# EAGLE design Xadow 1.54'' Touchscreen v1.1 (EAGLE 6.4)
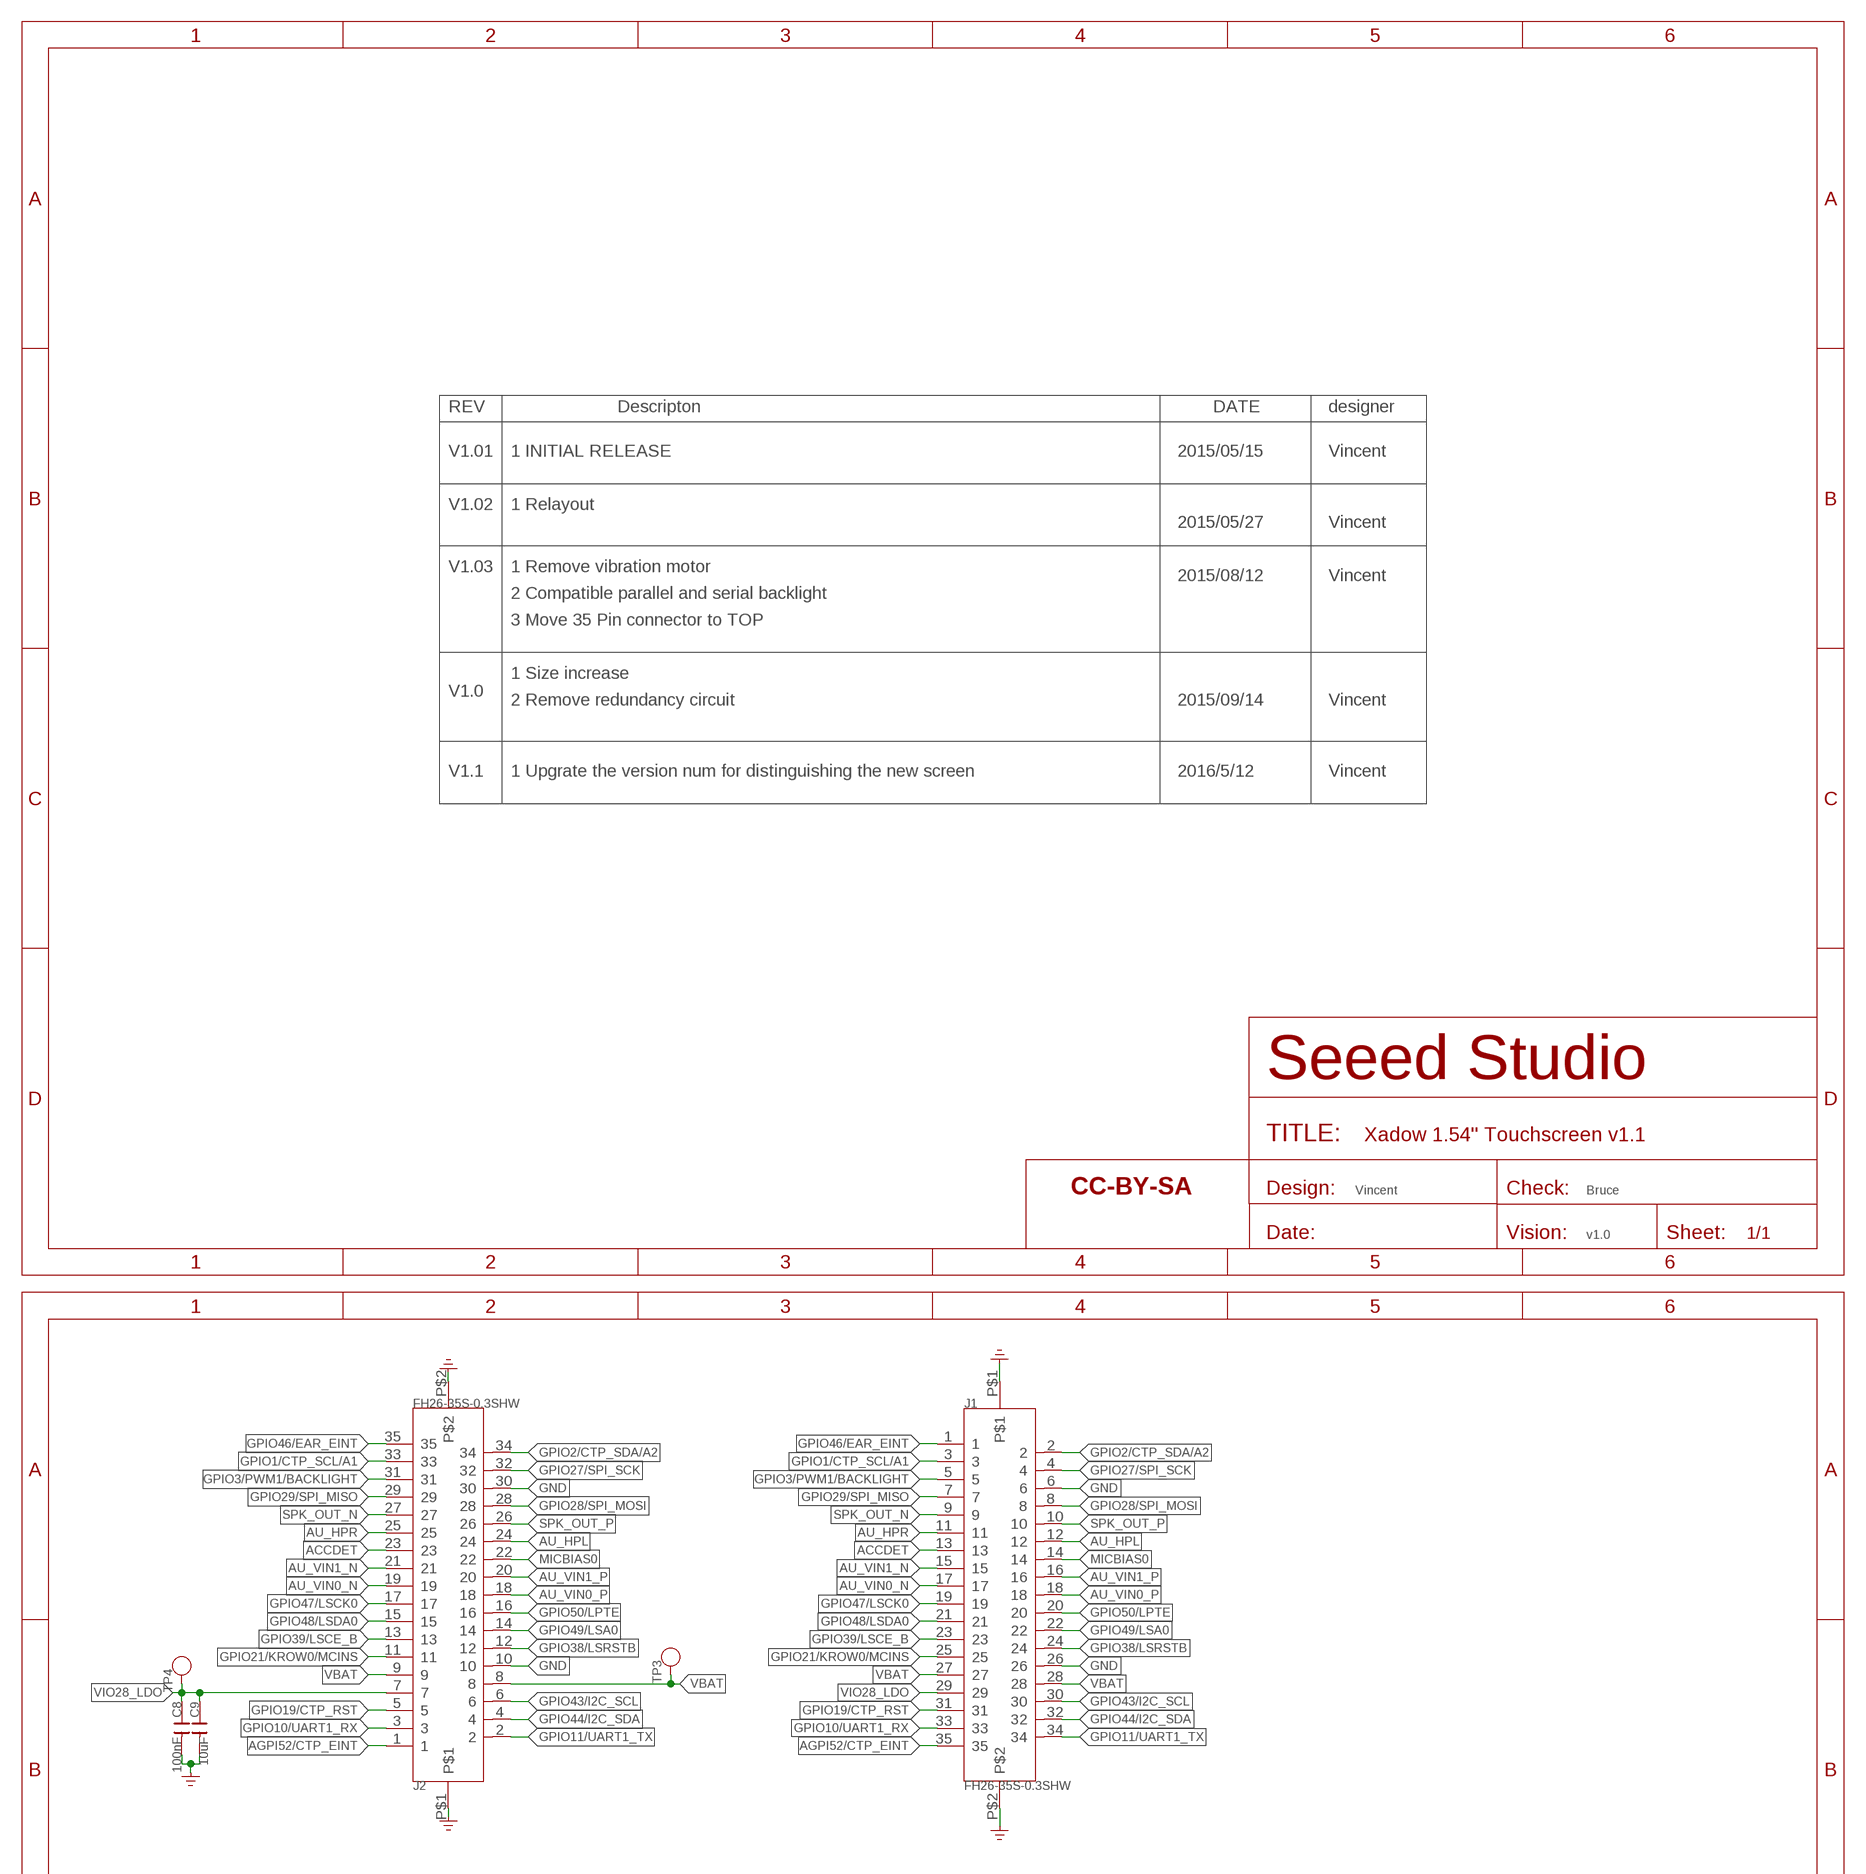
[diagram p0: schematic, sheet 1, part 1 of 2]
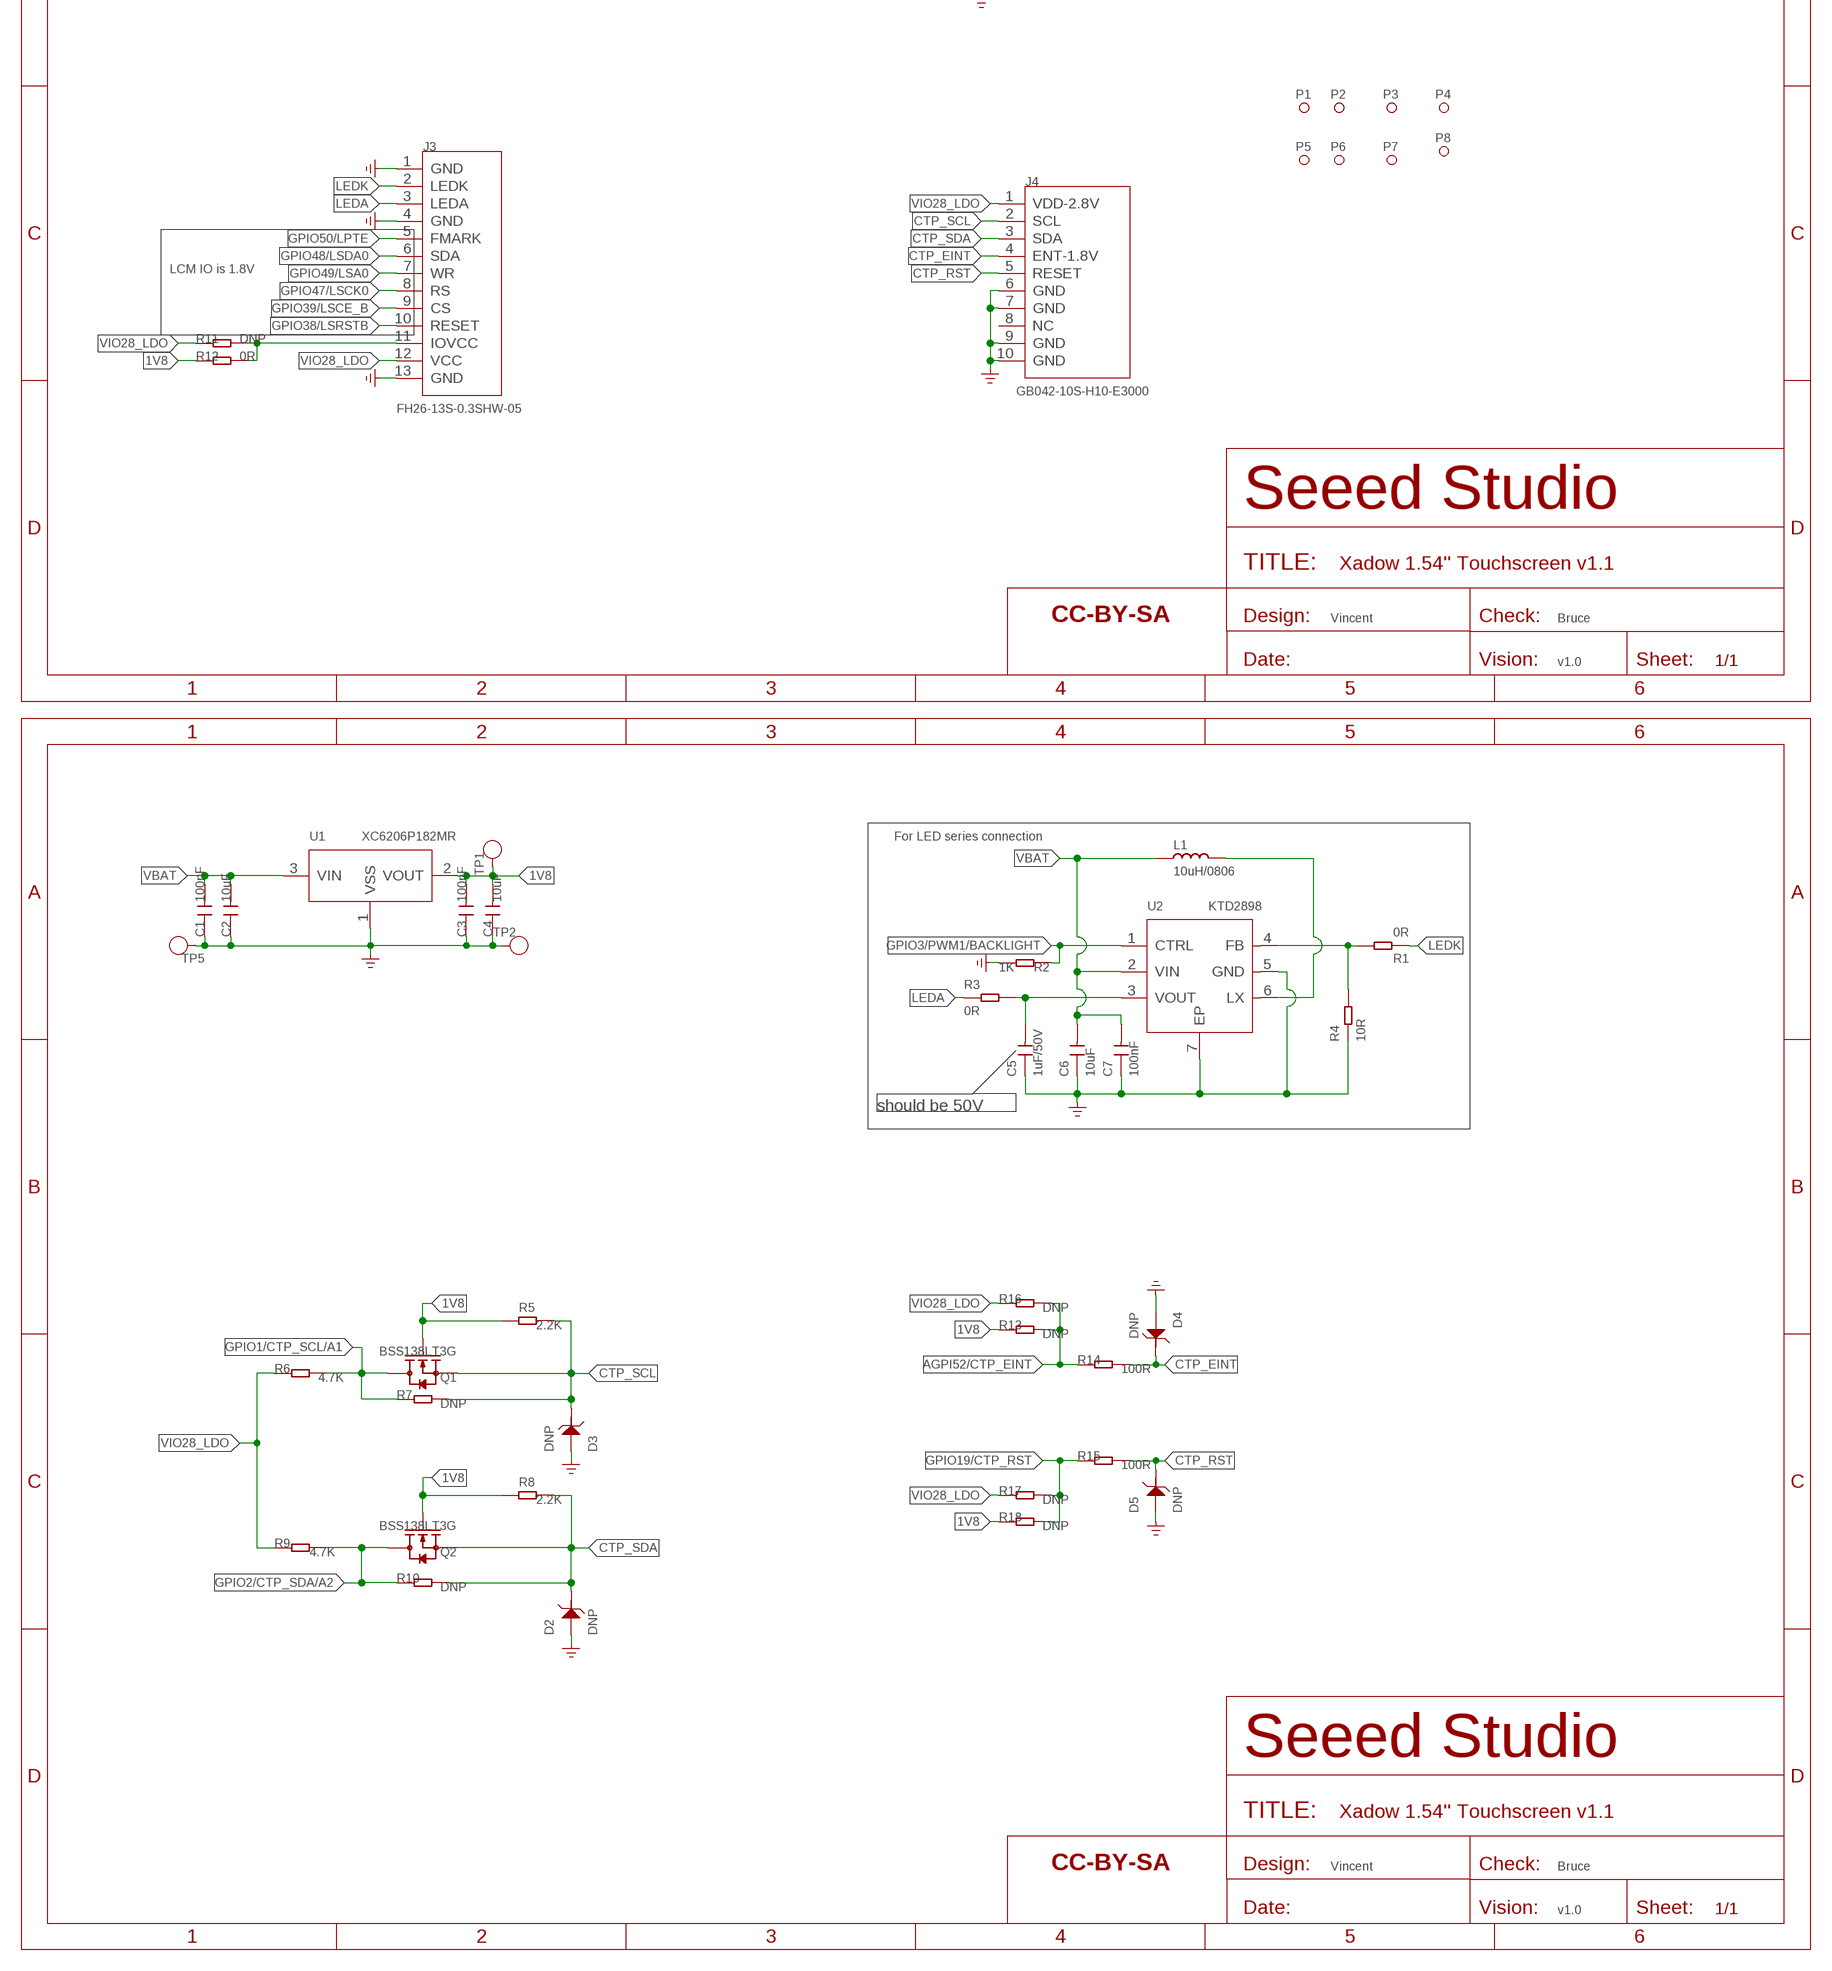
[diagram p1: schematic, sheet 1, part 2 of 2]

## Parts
C1  100nF  CAP-0402  [C0402]
C2  10uF  CAP-0603  [C0603]
C3  100nF  CAP-0402  [C0402]
C4  10uF  CAP-0603  [C0603]
C5  1uF/50V  CAP-0603  [C0603]
C6  10uF  CAP-0603  [C0603]
C7  100nF  CAP-0402  [C0402]
C8  100nF  CAP-0402  [C0402]
C9  10uF  CAP-0603  [C0603]
D2  DNP  D-ESD-2P'DF2S6.8FS'  [SOD-923]
D3  DNP  D-ESD-2P'DF2S6.8FS'  [SOD-923]
D4  DNP  D-ESD-2P'DF2S6.8FS'  [SOD-923]
D5  DNP  D-ESD-2P'DF2S6.8FS'  [SOD-923]
FR1  SEEEDSTUDIO-OPEN-SCH-FRAME  [SEEEDSTUDIO-PCB-FRAME]
FR2  SEEEDSTUDIO-OPEN-SCH-FRAME  [SEEEDSTUDIO-PCB-FRAME]
FR3  SEEEDSTUDIO-OPEN-SCH-FRAME  [SEEEDSTUDIO-PCB-FRAME]
J1  FH26-35S-0.3SHW  FPC-CONNECTER-35P(FH26W-35S-0.3SHW(10))  [FPC35-SMD-0.3(FH26W)]
J2  FH26-35S-0.3SHW  FPC-CONNECTER-35P(FH26W-35S-0.3SHW(10))  [FPC35-SMD-0.3(FH26W)]
J3  FH26-13S-0.3SHW-05  [13P-SMD-FH26-13S-0.3HW]
J4  GB042-10S-H10-E3000  [10P-SMD-GB042-10S-H10]
L1  10uH/0806  INDUCTOR/FERRITE-BEAD'0806'  [L0806]
P1  MARK-1.0'ANNULAR'  [ROUND-MARK-1.0]
P2  MARK-1.0'ANNULAR'  [ROUND-MARK-1.0]
P3  MARK-1.0'ANNULAR'  [ROUND-MARK-1.0]
P4  MARK-1.0'ANNULAR'  [ROUND-MARK-1.0]
P5  MARK-1.0'ANNULAR'  [ROUND-MARK-1.0]
P6  MARK-1.0'ANNULAR'  [ROUND-MARK-1.0]
P7  MARK-1.0'ANNULAR'  [ROUND-MARK-1.0]
P8  MARK-1.0'ANNULAR'  [ROUND-MARK-1.0]
Q1  BSS138LT3G  MOSFET-N'SOT23'  [SOT-23]
Q2  BSS138LT3G  MOSFET-N'SOT23'  [SOT-23]
R1  0R  RES-0402  [R0402]
R2  1K  RES-0402  [R0402]
R3  0R  RES-0402  [R0402]
R4  10R  RES-0402  [R0402]
R5  2.2K  RES-0402  [R0402]
R6  4.7K  RES-0402  [R0402]
R7  DNP  RES-0402  [R0402]
R8  2.2K  RES-0402  [R0402]
R9  4.7K  RES-0402  [R0402]
R10  DNP  RES-0402  [R0402]
R11  DNP  RES-0402  [R0402]
R12  0R  RES-0402  [R0402]
R13  DNP  RES-0402  [R0402]
R14  100R  RES-0402  [R0402]
R15  100R  RES-0402  [R0402]
R16  DNP  RES-0402  [R0402]
R17  DNP  RES-0402  [R0402]
R18  DNP  RES-0402  [R0402]
TP1  TEST-POINT'4545'  [TP-D45MIL]
TP2  TEST-POINT'4545'  [TP-D45MIL]
TP3  TEST-POINT'4545'  [TP-D45MIL]
TP4  TEST-POINT'4545'  [TP-D45MIL]
TP5  TEST-POINT'4545'  [TP-D45MIL]
U1  XC6206P182MR  PMIC-XC6206PMR  [SOT-23]
U2  KTD2898  [6P-SMD-KTD2898]

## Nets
1V8: C3.2 C4.2 Q1.1(G) Q2.1(G) R5.1 R8.1 R12.1 R13.1 R18.1 TP1.T U1.2(VOUT)
ACCDET: J1.13 J2.23
AGPI52/CTP_EINT: J1.35 J2.1 R13.2 R14.1 R16.2
AU_HPL: J1.12 J2.24
AU_HPR: J1.11 J2.25
AU_VIN0_N: J1.17 J2.19
AU_VIN0_P: J1.18 J2.18
AU_VIN1_N: J1.15 J2.21
AU_VIN1_P: J1.16 J2.20
CTP_EINT: D4.1 J4.4(ENT-1.8V) R14.2
CTP_RST: D5.1 J4.5(RESET) R15.2
CTP_SCL: D3.1 J4.2(SCL) Q1.2(S) R5.2 R7.2
CTP_SDA: D2.1 J4.3(SDA) Q2.2(S) R8.2 R10.2
GND: C1.1 C2.1 C3.1 C4.1 C5.1 C6.1 C7.1 C8.2 C9.2 D2.2 D3.2 D4.2 D5.2 J1.6 J1.26 J1.P$1 J1.P$2 J2.10 J2.30 J2.P$1 J2.P$2 J3.1(GND) J3.4(GND) J3.13(GND) J4.6(GND) J4.7(GND) J4.9(GND) J4.10(GND) R2.1 R4.1 TP2.T TP5.T U1.1(VSS) U2.5(GND) U2.7(EP) ; supply symbol labelled GND_POWER
GPIO1/CTP_SCL/A1: J1.3 J2.33 Q1.3(D) R6.2 R7.1
GPIO2/CTP_SDA/A2: J1.2 J2.34 Q2.3(D) R9.2 R10.1
GPIO3/PWM1/BACKLIGHT: J1.5 J2.31 R2.2 U2.1(CTRL)
GPIO10/UART1_RX: J1.33 J2.3
GPIO11/UART1_TX: J1.34 J2.2
GPIO19/CTP_RST: J1.31 J2.5 R15.1 R17.2 R18.2
GPIO21/KROW0/MCINS: J1.25 J2.11
GPIO27/SPI_SCK: J1.4 J2.32
GPIO28/SPI_MOSI: J1.8 J2.28
GPIO29/SPI_MISO: J1.7 J2.29
GPIO38/LSRSTB: J1.24 J2.12 J3.10(RESET)
GPIO39/LSCE_B: J1.23 J2.13 J3.9(CS)
GPIO43/I2C_SCL: J1.30 J2.6
GPIO44/I2C_SDA: J1.32 J2.4
GPIO46/EAR_EINT: J1.1 J2.35
GPIO47/LSCK0: J1.19 J2.17 J3.8(RS)
GPIO48/LSDA0: J1.21 J2.15 J3.6(SDA)
GPIO49/LSA0: J1.22 J2.14 J3.7(WR)
GPIO50/LPTE: J1.20 J2.16 J3.5(FMARK)
LEDA: J3.3(LEDA) R3.1
LEDK: J3.2(LEDK) R1.1
MICBIAS0: J1.14 J2.22
N$1: R1.2 R4.2 U2.4(FB)
N$2: C5.2 R3.2 U2.3(VOUT)
N$3: J3.11(IOVCC) R11.2 R12.2
N$5: L1.2 U2.6(LX)
SPK_OUT_N: J1.9 J2.27
SPK_OUT_P: J1.10 J2.26
VBAT: C1.2 C2.2 C6.2 C7.2 J1.27 J1.28 J2.8 J2.9 L1.1 TP3.T U1.3(VIN) U2.2(VIN)
VIO28_LDO: C8.1 C9.1 J1.29 J2.7 J3.12(VCC) J4.1(VDD-2.8V) R6.1 R9.1 R11.1 R16.1 R17.1 TP4.T
Unconnected: J4.8(NC)

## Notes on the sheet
- REV | Descripton | DATE | designer
- V1.01 | 1 INITIAL RELEASE | 2015/05/15 | Vincent
- V1.02 | 1 Relayout
- 2015/05/27 | Vincent
- V1.03 | 1 Remove vibration motor
- 2015/08/12 | Vincent
- 2 Compatible parallel and serial backlight
- 3 Move 35 Pin connector to TOP
- 1 Size increase
- V1.0
- 2 Remove redundancy circuit | 2015/09/14 | Vincent
- V1.1 | 1 Upgrate the version num for distinguishing the new screen | 2016/5/12 | Vincent
- Vincent | Bruce
- v1.0
- LCM IO is 1.8V
- Vincent | Bruce
- v1.0
- For LED series connection
- should be 50V
- Vincent | Bruce
- v1.0

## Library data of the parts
C1-C9 = Discrete-new:CAP: Ceramic Capacitors
D2-D5 = Discrete-new:D-ESD-2P: SOD-923:304060009;SOD-123:304060001
FR1-FR3 = moudle-new:SEEEDSTUDIO-OPEN-SCH-FRAME
J1 J2 = template:FPC-CONNECTER-35P(FH26W-35S-0.3SHW(10))
J3 = template:FH26-13S-0.3SHW-05
J4 = template:GB042-10S-H10-E3000
L1 = Discrete-new:INDUCTOR/FERRITE-BEAD
P1-P8 = Discrete-new:MARK-1.0; PARTNO: DNP
Q1 Q2 = Discrete-new:MOSFET-N
R1-R18 = Discrete-new:RES
TP1-TP5 = Discrete-new:TEST-POINT; PARTNO: DNP
U1 = IC-new:PMIC-XC6206P: LOW ESR Cap.Compatible Positive Voltage Regulators
U2 = template:KTD2898

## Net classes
0 default: width 0.076 mm, drill 0.102 mm, clearance 0.076 mm

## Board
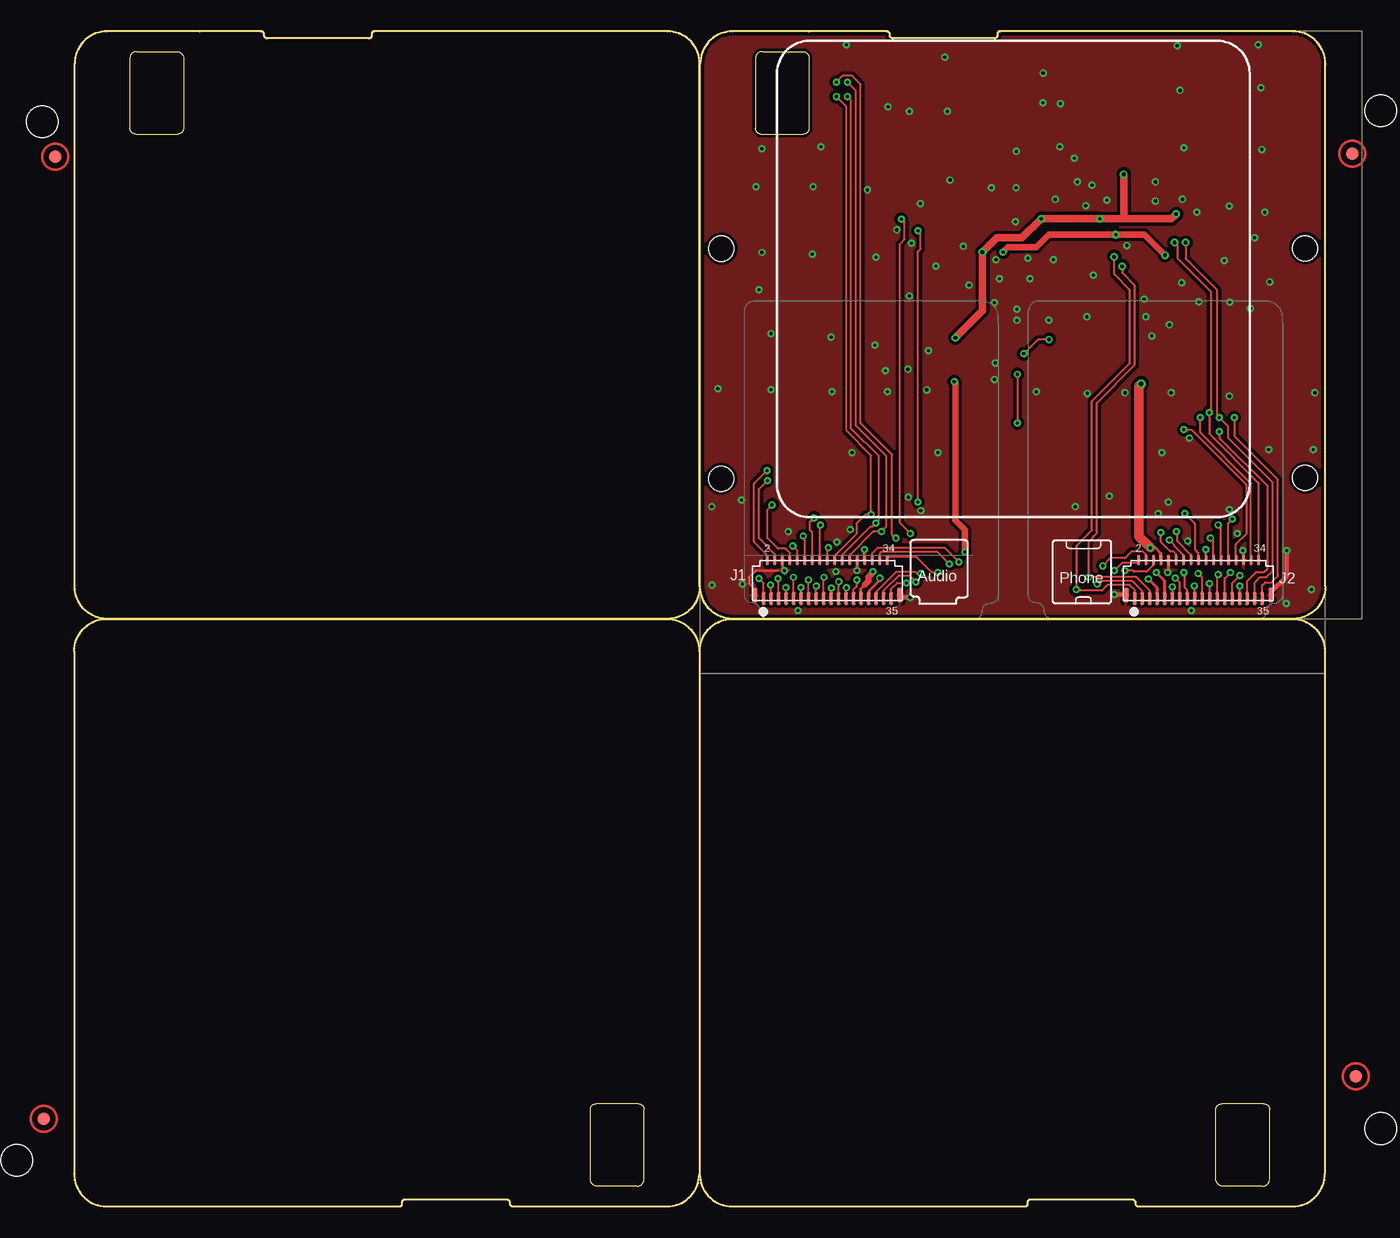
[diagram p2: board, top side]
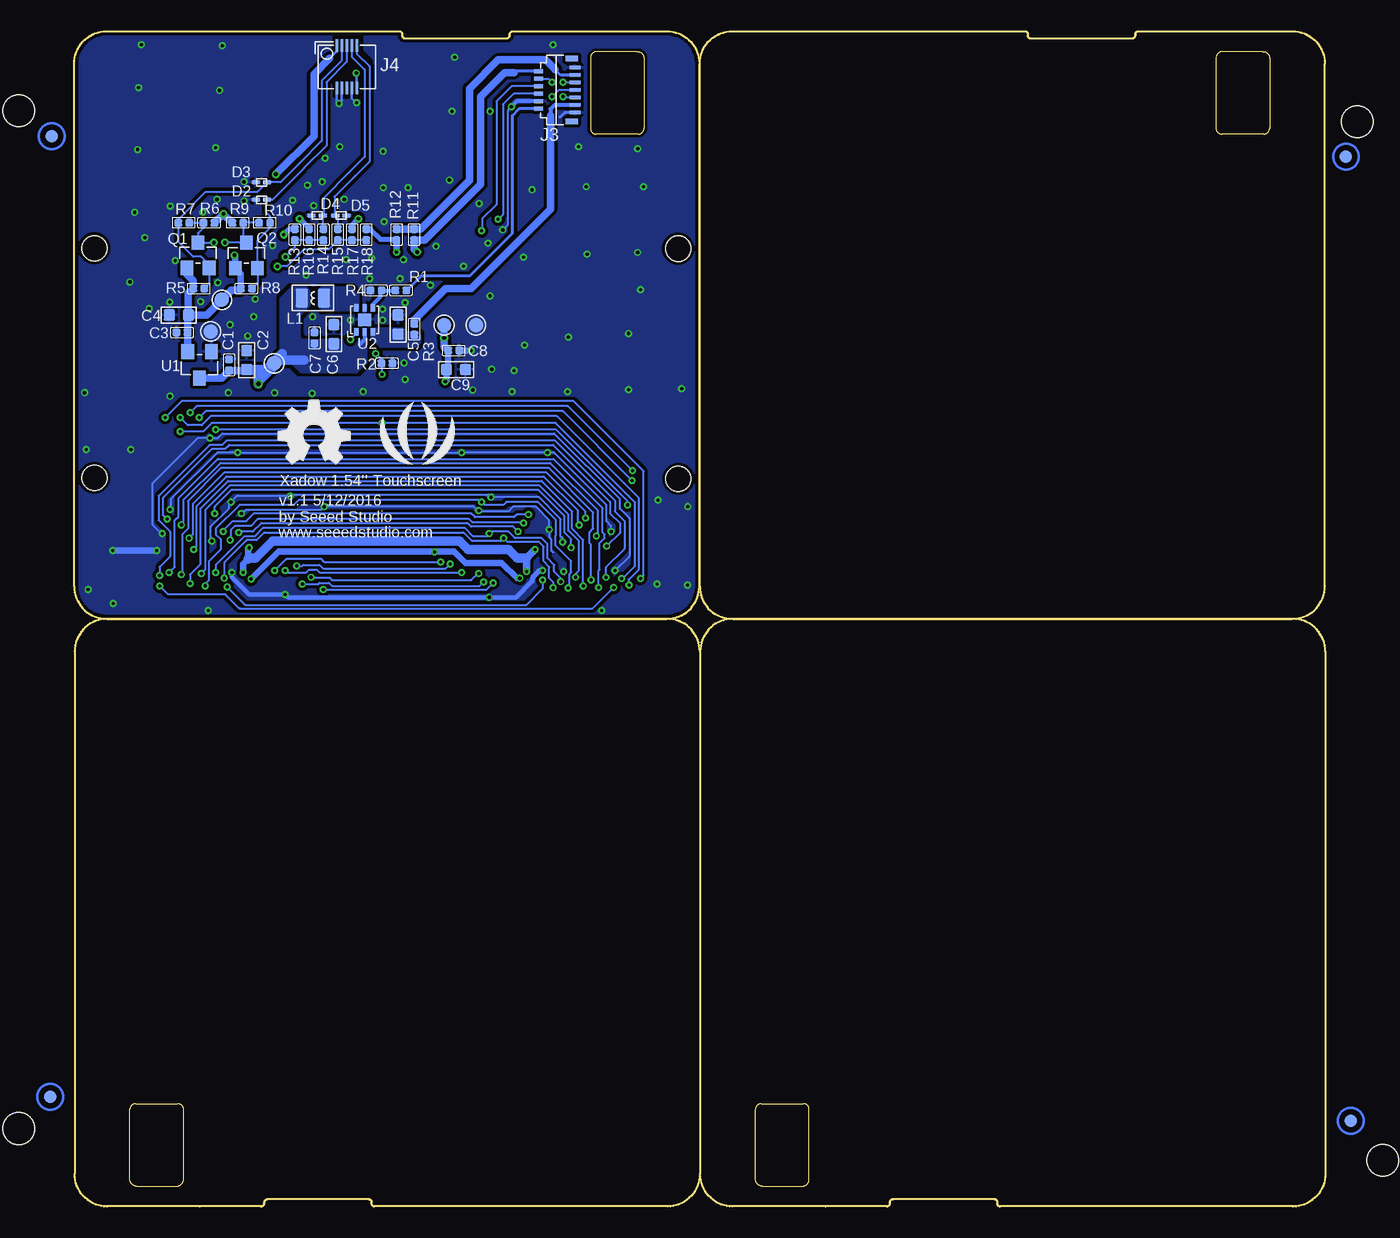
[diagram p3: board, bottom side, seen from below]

Size 100.08 x 94 mm. Coordinates in mm from the lower left corner, seen from the top.
Outline: 104 segments
Copper layers (1*16): Top 0.035mm / dielectric 1.5mm / Bottom 0.035mm
Design rules "SeeedStudio_2layer_DRU_no_angle_20140221 *": minimum track width 6mil, minimum drill 10mil, track to track 6mil, track to pad 6mil, pad to pad 6mil, via to via 6mil, smd to smd 0mil, copper to edge 10mil, drill to drill 10mil, minimum pad ring 10mil, minimum via ring 6mil, stop-mask expansion 2mil, vias tented up to drill 25mil, thermal gap 10mil
Holes 2.03 mm at 51.77,76.62 51.74,58.2 98.46,58.28 98.46,76.64
Holes 2.54 mm at -2.54,86.75 -4.57,3.69 104.52,6.23 104.52,87.64

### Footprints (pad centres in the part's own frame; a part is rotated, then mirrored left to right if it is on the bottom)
C0402 = smd 0.635 x 0.635: 1 0,0.445; 2 0,-0.445
C0603 = smd 0.889 x 0.889: 1 0,0.762; 2 0,-0.762
SOD-923 = smd 0.7 x 0.3: 1 -0.45,0; 2 0.45,0
FPC35-SMD-0.3(FH26W) = smd 0.3 x 1: 1 -5.1,-1.551; 3 -4.5,-1.551; 5 -3.9,-1.551; 7 -3.3,-1.551; 9 -2.7,-1.551; 11 -2.1,-1.551; 13 -1.5,-1.551; 15 -0.9,-1.551; 17 -0.3,-1.551; 19 0.3,-1.551; 21 0.9,-1.551; 23 1.5,-1.551; 25 2.1,-1.551; 27 2.7,-1.551; 29 3.3,-1.551; 31 3.9,-1.551; 33 4.5,-1.551; 35 5.1,-1.551 | smd 0.254 x 0.851: 2 -4.8,1.524; 4 -4.2,1.524; 6 -3.6,1.524; 8 -3,1.524; 10 -2.4,1.524; 12 -1.8,1.524; 14 -1.2,1.524; 16 -0.6,1.524; 18 0,1.524; 20 0.6,1.524; 22 1.2,1.524; 24 1.8,1.524; 26 2.4,1.524; 28 3,1.524; 30 3.6,1.524; 32 4.2,1.524; 34 4.8,1.524 | smd 0.4 x 1.15: P$1 5.8,-1.276; P$2 -5.8,-1.276
13P-SMD-FH26-13S-0.3HW = smd 0.3 x 0.85: 1 -1.8,-1.462; 3 -1.2,-1.462; 5 -0.6,-1.462; 7 0,-1.462; 9 0.6,-1.462; 11 1.2,-1.462; 13 1.8,-1.462 | smd 0.3 x 0.7: 2 -1.5,1.462; 4 -0.9,1.462; 6 -0.3,1.462; 8 0.3,1.462; 10 0.9,1.462; 12 1.5,1.462 | smd 0.45 x 1: 14 2.525,-1.188; 15 -2.525,-1.188
10P-SMD-GB042-10S-H10 = smd 0.23 x 1: 1 -0.8,1.7; 2 -0.4,1.7; 3 0,1.7; 4 0.4,1.7; 5 0.8,1.7; 6 0.8,-1.7; 7 0.4,-1.7; 8 0,-1.7; 9 -0.4,-1.7; 10 -0.8,-1.7
L0806 = smd 1.016 x 1.524: 1 -0.889,0; 2 0.889,0
ROUND-MARK-1.0 = smd 1.016 x 1.016: P$1 0,0
SOT-23 = smd 1.016 x 1.143: 1 -0.889,-1.016; 2 0.889,-1.016; 3 0,1.016
R0402 = smd 0.635 x 0.635: 1 0,0.445; 2 0,-0.445
TP-D45MIL = smd 1.143 x 1.143: T 0,0
SOT-23' = smd 1.016 x 1.2: 1 -0.95,-1.06; 2 0.95,-1.06; 3 0,1.06
6P-SMD-KTD2898 = smd 0.35 x 0.58: 1 -0.65,-0.96; 2 0,-0.96; 3 0.65,-0.96; 4 0.65,0.96; 5 0,0.96; 6 -0.65,0.96 | smd 1 x 1: 7 0,0

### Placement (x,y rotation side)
C1  87.68,67.31 0 bottom
C2  86.28,67.69 0 bottom
C3  91.45,69.91 90 bottom
C4  91.7,71.31 90 bottom
C5  74.17,70.54 0 bottom
C6  79.3,69.77 0 bottom
C7  80.85,69.47 0 bottom
C8  69.72,68.46 90 bottom
C9  69.54,66.94 90 bottom
D2  85.09,80.53 180 bottom
D3  85.09,81.92 180 bottom
D4  80.64,79.26 180 bottom
D5  78.74,79.26 0 bottom
FR1  not placed on the board
FR2  not placed on the board
FR3  not placed on the board
J1  60.24,50.17 0 top
J2  89.92,50.17 0 top
J3  61.47,89.3 90 bottom
J4  78.26,91.15 0 bottom
L1  80.98,72.66 0 bottom
P1  101.98,8.77 0 bottom
P2  -2.03,6.87 0 bottom
P3  -1.65,83.96 0 bottom
P4  101.85,85.61 0 bottom
P5  -2.41,6.99 0 top
P6  102.49,10.42 0 top
P7  102.23,84.21 0 top
P8  -1.52,83.96 0 top
Q1  90.17,76.08 0 bottom
Q2  86.3,76.08 0 bottom
R1  73.95,73.27 270 bottom
R2  75.06,67.45 270 bottom
R3  72.88,70.17 0 bottom
R4  75.93,73.27 90 bottom
R5  90.11,73.42 90 bottom
R6  89.29,78.69 270 bottom
R7  91.31,78.69 270 bottom
R8  86.3,73.42 90 bottom
R9  86.99,78.69 90 bottom
R10  84.84,78.69 90 bottom
R11  72.9,77.73 180 bottom
R12  74.3,77.73 180 bottom
R13  82.42,77.73 0 bottom
R14  80.14,77.73 180 bottom
R15  78.99,77.73 180 bottom
R16  81.28,77.73 0 bottom
R17  77.85,77.73 0 bottom
R18  76.71,77.73 0 bottom
TP1  88.27,72.53 0 bottom
TP2  89.15,69.99 0 bottom
TP3  84.07,67.45 0 bottom
TP4  70.48,70.5 0 bottom
TP5  67.94,70.5 0 bottom
U1  XC6206P182MR  [SOT-23']  90.04,67.32 180 bottom
U2  76.84,70.92 0 bottom
U$18  [OSHW_FILLX200_NOTEXT]  83.73,59.41 0 bottom
U$20  [SEEED-SILK-280*268MIL]  72.63,61.06 0 bottom

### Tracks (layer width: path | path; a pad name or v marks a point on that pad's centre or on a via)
1V8  (via drill 0.25 pad 0.51, 0.25 pad 0.61, 0.3)
  Top 0.508: v74.3,76.34 74.68,76.72 76.96,76.72 77.98,77.73 v83.31,77.73 85.6,77.73 v87.25,76.08
  Bottom 0.406: R13.1 82.87,78.18 v83.31,77.73 | R18.1 76.39,78.18 75.56,77.35 74.36,77.35 R12.1
  Bottom 0.508: R8.1 86.74,74.61 Q2.1 87.19,76.02 v87.25,76.08 | R12.1 v74.3,76.34
  Bottom 0.61: Q1.1 91.06,74.56 90.55,74.05 R5.1 90.94,73.03 C4.2 | C4.2 89.49,71.31 TP1.T 87.57,73.23 87.5,73.29 86.87,73.29 R8.1 | U1.2 90.99,69.9 C3.2 91,71.24 C4.2
ACCDET  (via drill 0.25 pad 0.51)
  Top 0.152: J2.23 91.42,50.48 v91.5,50.56 | J1.13 v58.74,50.12
  Bottom 0.152: v58.74,50.12 58.74,52.94 58.87,53.07 58.87,53.91 58.57,54.21 58.57,55.51 62.15,59.09 88.3,59.09 90.96,56.42 90.96,54.21 91.42,53.76 91.42,50.63 v91.5,50.56
AGPI52/CTP_EINT  (via drill 0.25 pad 0.51, 0.3)
  Top 0.152: J1.35 65.34,49.38 65.83,49.87 v66.57,49.87 | J2.1 84.82,49.31 84.41,49.72 82.66,49.72 82.2,49.26 80.22,49.26 v80.14,49.34 80.14,52.84 80.83,53.53 81.41,54.11 81.41,64.4 84.45,67.45 84.45,73.29 83.19,74.56 v83.19,75.96
  Bottom 0.152: v66.57,49.87 67.1,49.34 v80.14,49.34 | R14.1 R16.2 R13.2 82.42,76.72 v83.19,75.96
AU_HPL  (via drill 0.25 pad 0.51)
  Top 0.152: J1.12 58.44,53.5 v58.31,53.63 | J2.24 91.72,54.29 v91.5,54.52
  Bottom 0.152: v91.5,54.52 91.34,54.67 91.34,56.5 88.37,59.47 62,59.47 58.19,55.66 58.19,53.91 58.31,53.78 v58.31,53.63
AU_HPR  (via drill 0.25 pad 0.51)
  Top 0.152: J1.11 58.14,49.51 v58.13,49.52 | 92.03,48.63 J2.25 92.02,50.24 v92.49,50.71
  Bottom 0.152: v92.49,50.71 92.03,51.17 92.03,54.9 91.73,55.2 91.73,56.64 88.58,59.79 61.75,59.79 57.8,55.84 57.8,53.91 57.65,53.76 57.65,53.45 58.03,53.07 58.03,50.94 58.13,50.84 v58.13,49.52
AU_VIN0_N  (via drill 0.25 pad 0.51)
  Top 0.152: J1.17 59.94,50.31 v59.96,50.33 | J2.19 90.22,50.31 v89.9,50.63
  Bottom 0.152: v89.9,50.63 89.59,50.94 89.59,55.71 87.61,57.7 62.9,57.7 60.55,55.34 60.55,54.06 59.71,53.22 59.71,50.86 59.96,50.61 v59.96,50.33
AU_VIN0_P  (via drill 0.25 pad 0.51)
  Top 0.152: J1.18 60.24,52.61 v60.32,52.69 | J2.18 89.92,52.28 89.67,52.54 89.67,54.59 v88.83,55.43
  Bottom 0.152: v60.32,52.69 60.32,53.38 60.85,53.91 60.85,55.22 62.97,57.34 87.46,57.34 88.83,55.97 v88.83,55.43
AU_VIN1_N  (via drill 0.25 pad 0.51)
  Top 0.152: J1.15 59.34,49.6 v59.35,49.62 | J2.21 90.82,49.81 v90.81,49.82
  Bottom 0.152: v59.35,49.62 59.35,53.33 60.24,54.21 60.24,55.59 62.69,58.03 87.77,58.03 89.97,55.83 89.97,51.39 90.81,50.56 v90.81,49.82
AU_VIN1_P  (via drill 0.25 pad 0.51)
  Top 0.152: J2.20 90.52,52.52 v90.51,52.54 | J1.16 59.64,54.45 v59.68,54.49
  Bottom 0.152: v90.51,52.54 90.28,52.77 90.28,56.01 87.89,58.4 62.52,58.4 59.79,55.66 59.79,54.82 59.68,54.72 v59.68,54.49
CTP_EINT
  Bottom 0.152: J4.4 77.86,91.97 76.83,90.94 76.83,83.96 77.99,82.8 78.11,82.69 80.14,80.66 80.14,79.32 D4.1 80.19,78.24 R14.2
CTP_RST
  Bottom 0.152: J4.5 77.47,92.21 76.45,91.2 76.45,83.58 77.61,82.42 77.72,82.31 79.25,80.78 79.25,79.26 D5.1 arc90 78.99,79.06 R15.2
CTP_SCL
  Bottom 0.152: J4.2 78.67,91.65 80.26,90.05 80.26,85.23 82.04,83.45 82.17,83.32 83.57,81.92 D3.1 85.4,81.16 89.53,81.16 91.75,78.95 R7.2 91.75,77.16 90.55,75.96 89.92,75.96 89.28,75.32 Q1.2 89.28,73.8 R5.2
CTP_SDA
  Bottom 0.152: J4.3 78.27,91.54 79.88,89.93 79.88,84.85 81.66,83.07 81.72,83 84.2,80.53 D2.1 84.71,80.46 84.71,79.51 84.4,79.2 R10.2 84.4,78.3 85.41,77.29 Q2.2 85.41,73.87 R8.2
GND  (via drill 0.25, 0.25 pad 0.51)
  Top 0.152: J1.P$1 | 56.31,50.84 54.48,50.84 53.97,50.33 53.97,49.82 54.38,49.41 54.38,48.97 J1.P$2 | J1.6 56.64,51.03 v56.81,50.86
  Top 0.203: J2.30 93.52,52.42 v93.48,52.46
  Top 0.229: J2.10 87.52,50.77 v87.46,50.71
  Top 0.254: J1.26 62.6,51.66 v62.6,50.86
  Top 0.356: 95.72,48.88 J2.P$1 95.72,49.14 96.98,50.4 v96.98,52.46 | 66.06,48.88 J1.P$1 66.22,48.73 v66.87,48.73 | v83.19,48.96 84.07,48.96 J2.P$2
  Bottom 0.152: 82.73,56.88 v82.81,56.8 | v82.81,56.8 87.08,56.8 v87.53,56.35 87.69,56.2 87.69,55.81 89.14,54.37 89.14,53.38 89.06,53.3 v89.06,53.22 | v82.81,56.8 82.66,56.96 66.95,56.96 v66.72,56.73 62.91,56.73 61.16,54.98 61.16,53.6 61.01,53.45 v61.01,53.15 | v86.7,55.43 86.62,55.43 86.32,55.74 80.3,55.74 v80.07,55.97 79.99,56.04 68.17,56.04 67.79,55.66 v67.71,55.66 67.64,55.59 65.35,55.59 64.97,55.97 63.14,55.97 62.07,54.9 v62.07,54.14 62.07,53.53 61.92,53.38 61.92,52.46 61.77,52.31 | v93.02,53.83 93.1,53.83 93.78,54.52 93.78,57.87 90.2,61.45 v89.21,61.45 88.6,61.45 88.22,61.83 61.69,61.83 56.43,56.58 56.43,55.81 55.67,55.05 55.67,52 v56.81,50.86 | v57.12,53.98 57.12,54.44 57.5,54.82 57.5,56.12 61.69,60.31 v62.22,60.31 v69.08,60.31 v87,60.31 88.6,60.31 92.34,56.58 92.34,55.81 v92.41,55.74 | 65.11,87.94 65.41,87.64 65.41,78.5 v65.79,78.11
  Bottom 0.203: J4.7 77.86,88.66 v77.48,88.28 | J4.6 77.47,90.62 v77.5,90.66 | J4.10 79.06,88.41 v78.87,88.22 78.67,88.43 J4.9
  Bottom 0.254: v65.11,87.97 65.11,87.94 | J3.1 60.84,87.5 61.21,87.13 | 78.67,88.48 78.87,88.28
  Bottom 0.305: J3.4 64.68,88.4 v65.11,87.97
  Bottom 0.356: 63.44,50.02 64.74,48.73 v66.87,48.73 82.96,48.73 v83.19,48.96 86.08,48.96 87.46,50.33 v87.46,50.71
  Bottom 0.406: 63.44,50.02 63.44,50.25 62.83,50.86 v62.6,50.86
  Bottom 0.508: v96.98,52.46 v93.48,52.46 | C8.2 v68.33,68.46
  other vias: 75.39,70.88 77.96,70.9 73.69,67.47 73.62,66.15 66.81,72.83 66.67,66.96 68.19,65.31 53.46,49.79 64.89,66.86 65.04,65.19 64.05,68.89 64.14,75.93 60.55,69.53 60.62,65.19 51.48,65.41 54.77,73.34 59.04,76.16 55.75,69.83 55.75,65.34 54.54,81.57 59.11,81.57 63.46,81.32 55,84.62 59.72,84.77 61.78,92.92 69.63,91.93 69.86,87.59 70.06,82.1 75.37,84.39 78.82,84.77 75.34,81.49 73.36,81.49 81.41,81.7 88.22,92.85 88.45,89.27 88.75,84.69 95,84.54 94.93,89.49 94.7,92.92 92.39,80.02 95.23,79.51 95.61,73.95 92.01,75.65 80.25,81.95 82.61,80.48 81.52,74.48 76.97,65.16 87.74,65.08 99.24,65.08 88.58,73.9 99.12,60.54 95.54,60.54 98.97,49.34 51.02,49.72 51,55.99 53.39,56.5 94.42,77.48 66.96,77.05 60.93,50.78 89.36,47.66 57.88,47.66 81.01,71.16 75.39,71.77 94.09,71.82 92.44,72.32 85.58,72.58 84.06,65.08 81.03,65.03 76.44,74.2 96.96,48.22 85.71,71.16 87.61,70.52 55,76.31 66.81,87.59 67.7,80.22 71.13,76.79 92.41,64.81 86.19,69.63 71.58,73.7 73.62,72.3 74,74.2 73.74,75.73 68.92,75.22 78.32,75.73 76.28,75.85 89.97,72.37 86.49,80.43 86.49,81.95 89.8,79.54 79.99,83.86 78.47,80.55 75.29,78.78 88.65,80.55 80.91,80.05 84.21,76.87
  pour Top (isolate 0.254, rank 3): 98.55,95.77 60.83,95.77 59.31,94.24 51.94,94.24 49.4,92.59 49.28,84.85 49.28,48.91 51.44,46.75 98.04,46.75 100.84,49.54 100.84,93.48
  pour Bottom (isolate 0.254, rank 3): 99.57,95.13 80.9,95.13 79.5,93.74 79.5,88.78 79.25,88.53 76.96,88.53 76.07,89.42 76.07,91.7 76.83,92.47 76.83,94.75 76.58,95.01 51.94,95.01 50.04,93.1 50.04,48.52 51.44,47.13 99.06,47.13 100.33,48.4 100.33,94.37
GPIO1/CTP_SCL/A1  (via drill 0.25 pad 0.51, 0.3)
  Top 0.152: J2.33 94.42,49.9 94.85,50.33 95.36,50.33 95.87,50.84 95.87,57.92 92.31,61.48 92.31,62.39 v91.6,63.1 91.42,63.28 91.42,73.31 88.9,75.83 v88.9,77.1 | J1.3 55.74,49.67 v55.7,49.72
  Bottom 0.152: v91.6,63.1 90.99,62.49 89.87,62.49 89.16,63.2 61.47,63.2 54.91,56.64 54.91,50.94 55.7,50.15 v55.7,49.72 | R7.1 R6.2 89.73,78.3 90.17,77.86 Q1.3 v88.9,77.1 v88.91,77.09
GPIO2/CTP_SDA/A2  (via drill 0.25 pad 0.51, 0.3)
  Top 0.152: J2.34 94.72,57.87 90.79,61.81 v90.79,63.51 90.93,63.66 90.93,73.16 88.27,75.83 88.27,76.84 v88.01,77.1 | J1.2 55.44,52.08 54.38,53.15 54.38,57.82 v55.42,58.86
  Bottom 0.152: v90.79,63.51 90.28,64.02 60.57,64.02 v55.42,58.86 | R10.1 R9.2 86.54,77.34 Q2.3 v88,77.09 v88.01,77.1
GPIO3/PWM1/BACKLIGHT  (via drill 0.25, 0.25 pad 0.51)
  Top 0.152: J2.31 93.82,50.01 94.55,50.73 95.16,50.73 95.46,51.04 95.46,57.62 91.6,61.48 v91.6,61.99 | J1.5 56.34,50.19 v56.31,50.23 | v75.44,66.56 v75.44,62.67 | v77.98,69.35 77.09,69.35 v75.95,68.21
  Bottom 0.152: v91.6,61.99 89.77,61.99 89.08,62.67 v75.44,62.67 61.57,62.67 55.73,56.84 55.21,56.32 55.21,51.24 56.23,50.23 v56.31,50.23 | U2.1 77.49,69.84 v77.98,69.35 | v75.95,68.21 75.5,67.77 R2.2 75.5,66.62 v75.44,66.56
GPIO10/UART1_RX  (via drill 0.25 pad 0.51)
  Top 0.152: J1.33 64.74,49.26 65.97,50.48 66.8,50.48 v67.33,49.95 | J2.3 85.42,49.24 84.64,50.02 82.05,50.02 v81.82,49.79
  Bottom 0.152: v81.82,49.79 80.53,49.79 80.45,49.87 79.69,49.87 79.46,49.64 67.64,49.64 v67.33,49.95 67.41,49.87
GPIO11/UART1_TX  (via drill 0.25)
  Top 0.152: J1.34 65.04,51.85 65.2,52 67.33,52 68.62,50.71 v69.08,50.71 | J2.2 85.12,51.65 84.94,51.47 83.8,51.47 v83.19,50.86
  Bottom 0.152: v83.19,50.86 83.12,50.86 82.96,50.71 81.52,50.71 81.29,50.94 80.68,50.94 80.45,50.71 v69.08,50.71
GPIO19/CTP_RST  (via drill 0.25 pad 0.51, 0.3)
  Top 0.152: J1.31 64.14,49.16 65.77,50.78 67.25,50.78 67.41,50.63 v67.71,50.63 | J2.5 86.02,49.25 84.94,50.33 v81.14,50.33 81.14,53.15 81.52,53.53 81.52,53.59 81.79,53.86 81.79,64.27 84.84,67.32 84.84,73.67 83.82,74.69 v83.82,75.19
  Bottom 0.152: v81.14,50.33 81.06,50.25 79.61,50.25 79.46,50.1 68.32,50.1 67.79,50.63 v67.71,50.63 | v83.82,75.19 83.06,75.19 81.66,76.59 79.69,76.59 R15.1 R17.2 R18.2
GPIO21/KROW0/MCINS  (via drill 0.25 pad 0.51)
  Top 0.152: J1.25 62.34,49.38 62.6,49.64 v62.6,50.1 | v87.84,49.56 87.84,48.64 J2.11
  Bottom 0.152: v62.6,50.1 62.6,49.41 63.9,48.12 86.39,48.12 v87.84,49.56
GPIO27/SPI_SCK  (via drill 0.25 pad 0.51)
  Top 0.152: J2.32 94.12,57.84 90.08,61.88 v90.08,63.1 | J1.4 56.04,52.16 54.76,53.45 54.76,57.39 v55.44,58.07
  Bottom 0.152: v90.08,63.1 89.57,63.61 60.98,63.61 v55.44,58.07
GPIO28/SPI_MOSI  (via drill 0.25 pad 0.51)
  Top 0.152: J2.28 92.92,52.97 93.78,53.83 93.78,57.72 89.36,62.14 v88.75,62.14 | J1.8 57.24,52.26 56.89,52.61 56.28,52.61 55.44,53.45 55.44,55.74 v55.82,56.12
  Bottom 0.152: v55.82,56.12 55.82,56.43 61.53,62.14 v88.75,62.14
GPIO29/SPI_MISO  (via drill 0.25 pad 0.51)
  Top 0.152: J2.29 v93.22,49.61 v93.22,49.62 | J1.7 56.94,49.49 v56.92,49.52
  Bottom 0.152: v93.22,49.62 92.64,49.03 arc-45 92.46,48.96 87.99,48.96 86.92,47.89 arc-45 86.74,47.81 58.62,47.81 v56.92,49.52
GPIO38/LSRSTB  (via drill 0.25, 0.25 pad 0.51)
  Top 0.152: J1.24 62.07,51.73 62.07,52.16 63.9,53.98 v64.59,53.98 64.97,54.37 64.97,60.01 62.53,62.44 62.53,89.25 v61.85,89.93 | J2.12 88.12,52.18 87.92,52.38 87.69,52.38 86.93,53.15 v86.93,53.91
  Bottom 0.152: v86.93,53.91 86.85,53.98 85.78,53.98 85.1,54.67 68.62,54.67 68.32,54.37 64.97,54.37 v64.59,53.98 | J3.10 62.12,90.2 v61.85,89.93
GPIO39/LSCE_B  (via drill 0.25, 0.25 pad 0.51)
  Top 0.152: J2.13 88.42,49.9 v88.07,50.25 | v65.73,53.45 65.42,53.76 65.42,60.16 62.91,62.67 62.91,89.75 62.23,90.43 61.47,90.43 v60.96,89.93 | J1.23 61.74,49.47 v61.77,49.49
  Bottom 0.152: v88.07,50.25 88.07,51.49 86.26,53.3 85.48,53.3 84.87,53.91 68.93,53.91 68.24,53.22 65.96,53.22 v65.73,53.45 | 65.65,53.38 v65.73,53.45 | v65.73,53.45 65.42,53.15 62.91,53.15 62.53,52.77 62.53,51.62 62.07,51.17 62.07,50.25 61.77,49.95 v61.77,49.49 | J3.9 60.94,89.9 v60.96,89.93
GPIO43/I2C_SCL  (via drill 0.25, 0.25 pad 0.51)
  Top 0.152: J1.30 63.84,52.25 64.28,52.69 69.62,52.69 v70.76,51.55 | J2.6 86.32,51.33 85.78,50.78 84.79,50.78 84.72,50.86 v84.03,50.86
  Bottom 0.152: v84.03,50.86 83.12,51.77 80.3,51.77 80.07,51.55 v70.76,51.55
GPIO44/I2C_SDA  (via drill 0.25, 0.25 pad 0.51)
  Top 0.152: J1.32 64.44,52.24 64.59,52.38 69.01,52.38 v70,51.39 | J2.4 85.72,52.14 85.48,52.38 84.56,52.38 84.03,51.85 82.89,51.85 v82.28,51.24
  Bottom 0.152: v82.28,51.24 81.82,51.24 81.74,51.32 80.45,51.32 80.14,51.01 70.38,51.01 v70,51.39
GPIO46/EAR_EINT  (via drill 0.25 pad 0.51)
  Top 0.152: J2.35 95.02,49.69 95.26,49.92 95.77,49.92 96.27,50.43 96.27,58.12 92.79,61.61 v92.79,63.1 | J1.1 55.14,49.87 v54.78,50.23
  Bottom 0.152: v92.79,63.1 91.47,64.42 60.14,64.42 54.53,58.81 54.53,50.48 v54.78,50.23
GPIO47/LSCK0  (via drill 0.25 pad 0.51)
  Top 0.152: J2.17 89.62,49.61 v89.59,49.64 | J1.19 60.54,49.43 v60.57,49.46 | v67.48,56.35 67.48,76.38 67.69,76.59 67.69,77.83 v67.48,78.04
  Bottom 0.152: v89.59,49.64 89.59,49.79 89.29,50.1 89.29,51.62 88.37,52.54 88.37,53.38 88.75,53.76 88.75,54.21 86.85,56.12 82.51,56.12 82.12,56.5 67.64,56.5 v67.48,56.35 67.25,56.12 65.73,56.12 65.5,56.35 62.99,56.35 61.54,54.9 61.54,53.68 61.55,53.67 61.55,52.86 60.32,51.62 60.32,50.71 60.47,50.56 60.47,49.56 v60.57,49.46 | J3.8 65.09,89.6 66.29,88.4 66.29,80.15 67.44,79 67.44,78.08 v67.48,78.04
GPIO48/LSDA0  (via drill 0.25 pad 0.51)
  Top 0.152: J1.21 61.14,49.55 61.16,49.56 v61.16,49.97 | J2.15 89.02,49.3 88.83,49.49 88.83,50.63 v88.75,50.71 | v66.87,53.83 66.03,54.67 66.03,76.97 66.42,77.35 66.42,78.71 v66.16,78.97
  Bottom 0.152: v88.75,50.71 88.75,51.33 87.77,52.31 87.76,52.31 86.47,53.6 85.63,53.6 84.94,54.29 68.85,54.29 68.17,53.6 67.1,53.6 v66.87,53.83 66.72,53.98 65.35,53.98 64.81,53.45 62.68,53.45 62.22,52.99 62.22,51.85 61.69,51.32 61.69,50.78 61.16,50.25 v61.16,49.97 | J3.6 64.93,89 65.79,88.15 65.79,79.34 v66.16,78.97
GPIO49/LSA0  (via drill 0.25, 0.25 pad 0.51)
  Top 0.152: J1.22 61.46,51.72 61.46,52.16 63.67,54.37 63.83,54.37 v64.13,54.67 64.36,54.9 64.36,60.01 62.15,62.22 62.15,88.48 v61.85,88.78 | J2.14 88.72,52.11 87.99,52.84 87.99,52.92 v87.61,53.3
  Bottom 0.152: v87.61,53.3 87.53,53.38 87.53,54.13 87.22,54.44 85.94,54.44 85.4,54.98 68.47,54.98 68.24,54.75 64.21,54.75 v64.13,54.67 | J3.7 61.33,89.3 v61.85,88.78
GPIO50/LPTE  (via drill 0.25, 0.25 pad 0.51)
  Top 0.152: J1.20 60.84,52.07 62.6,53.83 62.6,54.67 63.29,55.36 v63.75,55.36 63.75,60.08 61.77,62.06 61.77,87.98 v60.96,88.78 | J2.16 89.32,52.12 88.22,53.22 88.22,53.91 v88.14,53.98
  Bottom 0.152: v63.75,55.36 64.66,55.36 64.89,55.13 68.02,55.13 68.32,55.43 85.71,55.43 86.32,54.82 87.38,54.82 88.14,54.06 v88.14,53.98 | J3.5 60.88,88.7 v60.96,88.78
LEDA
  Bottom 0.305: J3.3 61.64,88.1 61.98,87.77 61.98,87.26
  Bottom 0.61: R3.1 72.88,70.89 70.36,73.42 68.33,73.42 61.98,79.77 61.98,87.26
LEDK
  Bottom 0.254: J3.2 64.48,87.8 65.02,87.26 65.02,77.86 68.45,74.43 72.34,74.43 R1.1
MICBIAS0  (via drill 0.25 pad 0.51)
  Top 0.152: J2.22 91.12,53.22 v90.89,53.45 | J1.14 59.04,53.89 58.87,54.06 58.87,54.77 v59.18,55.08
  Bottom 0.152: v59.18,55.08 59.18,55.59 62.33,58.74 88.04,58.74 90.58,56.2 90.58,53.76 v90.89,53.45
N$1
  Bottom 0.305: U2.4 76.19,72.15 75.56,72.78 75.56,73.19 R4.2 R1.2
N$2
  pour Bottom (isolate 0.254, no thermals): 76.33,70.24 73.79,70.24 73.53,69.99 72.64,69.99 72.39,69.73 72.39,69.1 72.77,68.72 75.56,68.72 76.33,69.48
N$3
  Bottom 0.254: J3.11 61.16,90.5 61.72,91.07
  Bottom 0.61: R12.2 R11.2 72.38,78.18 68.45,82.11 68.45,89.42 66.17,91.7 62.36,91.7 61.72,91.07 61.59,90.94
N$5
  pour Bottom (isolate 0.254, no thermals): 80.26,73.54 77.98,73.54 77.34,72.91 77.34,71.77 77.47,71.64 80.14,71.64 80.52,72.02 80.52,73.29
SPK_OUT_N  (via drill 0.25 pad 0.51)
  Top 0.152: J1.9 57.54,50.31 v57.52,50.33 | J2.27 92.62,49.85 v93.25,50.48
  Bottom 0.152: v93.25,50.48 93.25,51.17 92.41,52 92.41,53.98 93.33,54.9 93.33,56.84 89.25,60.92 88.22,60.92 87.84,61.3 61.64,61.3 56.81,56.48 56.81,55.59 56.07,54.84 56.07,52.6 57.52,51.14 v57.52,50.33
SPK_OUT_P  (via drill 0.25, 0.25 pad 0.51)
  Top 0.152: J2.26 92.32,54.66 v92.64,54.98 | J1.10 57.84,52.45 v57.47,52.82
  Bottom 0.152: 57.27,53.02 v57.47,52.82 56.43,53.86 56.43,54.67 57.2,55.43 57.2,56.35 61.77,60.92 87.69,60.92 87.99,60.61 89.03,60.61 92.95,56.7 92.95,55.28 v92.64,54.98
VBAT  (via drill 0.25, 0.25 pad 0.51, 0.38)
  Top 0.229: J1.27 62.94,49.45 63.24,49.75 | J2.9 87.22,50.03 v86.55,50.71
  Top 0.254: J2.8 86.93,52.23 86.47,52.69 v86.09,52.69 | J1.28 63.22,51.73 v63.22,52.54
  Top 0.508: 63.24,49.75 63.52,50.02 63.52,50.33 63.9,50.71 v63.9,50.78
  Top 0.762: v86.09,52.69 85.17,53.6 85.17,65.62 v85.34,65.8
  Bottom 0.305: U2.2 76.84,69.34 77.22,68.97
  Bottom 0.508: v86.09,52.69 86.16,52.61 86.16,51.77 86.55,51.39 v86.55,50.71
  Bottom 0.61: v63.9,50.78 63.9,51.85 v63.22,52.54 | U1.3 88.29,66.26 C1.2 86.34,66.87 C2.2 85.86,66.93 | TP3.T 84.14,67.51
  Bottom 0.762: 63.9,51.85 64.66,51.85 65.35,52.54 68.55,52.54 69.23,53.22 84.18,53.22 85.55,51.85 86.09,51.85 86.16,51.77 | 81.66,67.7 83.57,67.7 85.34,65.92 v85.34,65.8 85.34,66.56 85.6,66.81 | 85.86,66.93 84.72,66.93 84.14,67.51 83.44,68.21
  pour Bottom (isolate 0.254, no thermals): 82.68,73.54 81.53,73.54 81.28,73.29 81.28,72.02 82.04,71.26 82.04,69.48 81.92,69.35 78.61,69.35 78.11,68.84 77.72,68.84 77.22,69.35 76.96,69.35 76.71,69.1 76.71,67.45 77.47,66.69 81.92,66.69 83.57,68.34 83.57,72.65
VIO28_LDO  (via drill 0.25, 0.25 pad 0.51, 0.25 pad 0.61, 0.3, 0.3 pad 0.61)
  Top 0.229: J2.7 86.62,49.49 v85.94,50.17
  Top 0.254: J1.29 63.6,48.68 63.6,49.26 64.43,50.1 v64.43,50.25
  Top 0.508: v71.25,52.33 71.25,54.11 70.48,54.87 70.48,65.88 v70.39,65.97
  Top 0.61: v70.48,69.48 72.64,71.64 v72.64,76.34 73.79,77.48 75.82,77.48 v77.34,79 v82.04,79 83.95,79 | 83.95,79 87.76,79 v88.14,79.38 | v83.95,82.56 83.95,79
  Bottom 0.254: J4.1 79.06,92.4 79.63,91.83 | J3.12 64.78,90.8 64.9,90.69
  Bottom 0.406: R16.1 81.28,78.24 v82.04,79 | R17.1 77.85,78.5 v77.34,79
  Bottom 0.508: v85.94,50.17 83.72,52.38 71.2,52.38 | v64.43,50.25 64.66,50.25 65.88,51.47 68.78,51.47 69.69,52.38 71.2,52.38 | 71.2,52.38 v71.25,52.33 | v70.39,65.97 70.3,66.06 C9.1 70.16,67.08 C8.1
  Bottom 0.61: R9.1 v88.14,79.38 R6.1 | v72.64,76.34 72.9,76.59 R11.1 72.06,77.29 67.56,81.78 67.56,88.78 65.66,90.69 64.9,90.69 | C8.1 70.48,68.79 v70.48,69.48 TP4.T | v83.95,82.56 80.9,85.61 80.9,90.56 79.63,91.83

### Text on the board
tPlace: Audio | Phone
bPlace: Xadow 1.54'' Touchscreen | v1.1 5/12/2016 | by Seeed Studio | www.seeedstudio.com

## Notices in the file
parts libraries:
moudle-new: This work is licensed under the Creative Commons Attribution 4.0 International License.
To view a copy of this license,visit:
http://creativecommons.org/licenses/by-sa/4.0
moudle-new: CC-BY-SA
